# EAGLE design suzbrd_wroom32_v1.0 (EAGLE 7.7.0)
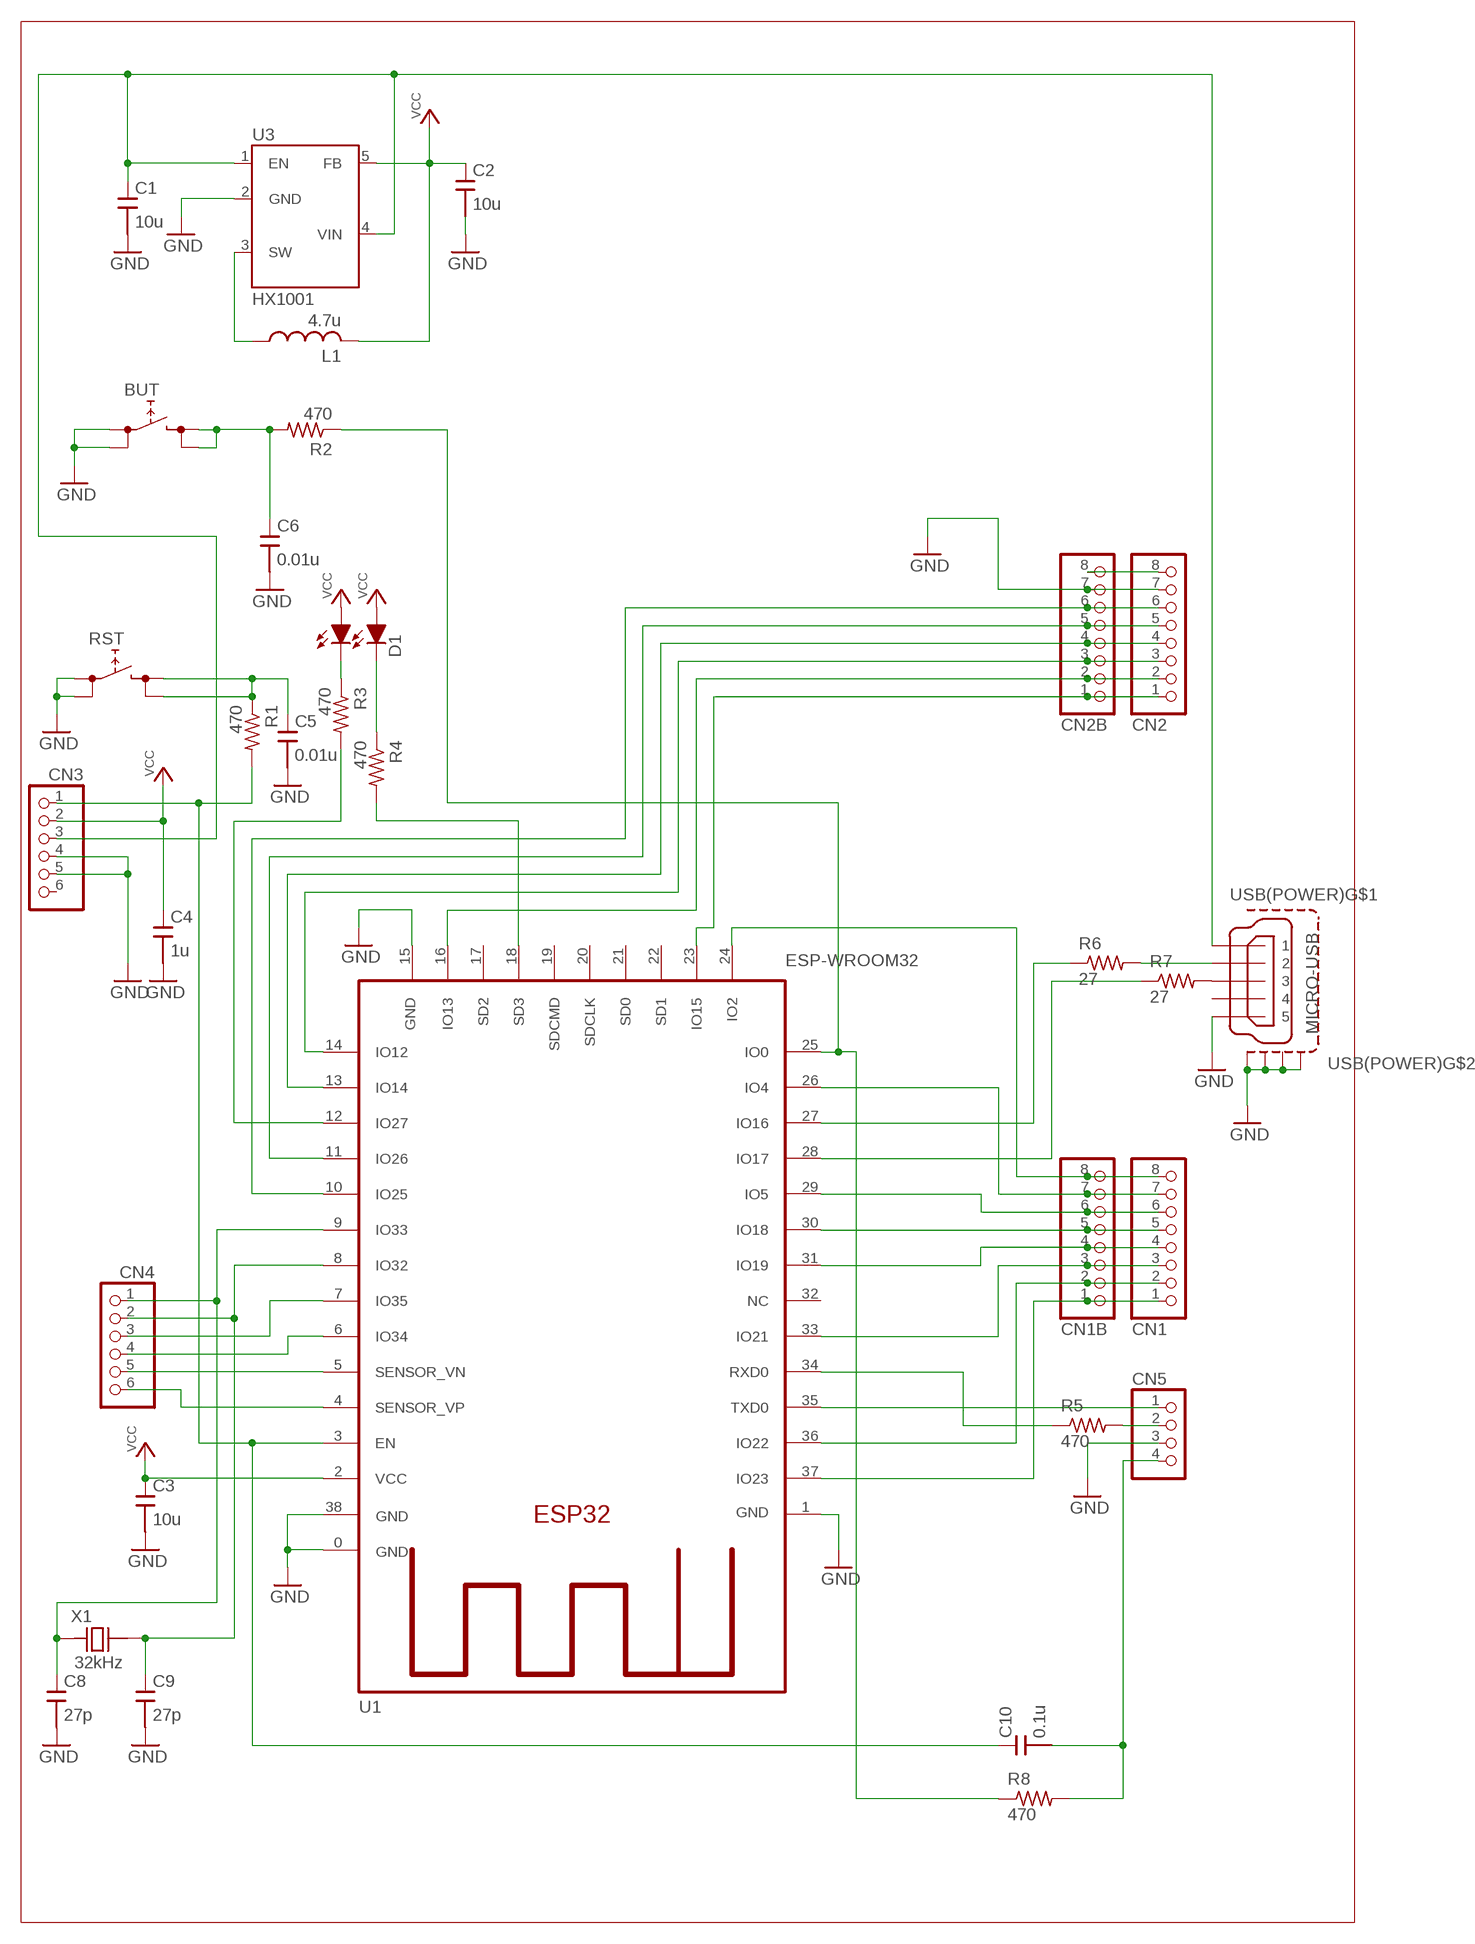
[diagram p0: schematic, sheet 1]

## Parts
BUT  TACTSWSMD+  [TACTSW/SMD+]
C1  10u  C/SMDC2012  [C2012]
C2  10u  C/SMDC2012  [C2012]
C3  10u  C/SMDC2012  [C2012]
C4  1u  C/SMDC2012  [C2012]
C5  0.01u  C/SMDC2012  [C2012]
C6  0.01u  C/SMDC2012  [C2012]
C8  27p  C/SMDC2012  [C2012]
C9  27p  C/SMDC2012  [C2012]
C10  0.1u  C/SMDC2012  [C2012]
CN1  PINHDR8  [PINHDR1X8]
CN1B  PINHDR81.0  [PINHDR1X8_1.0]
CN2  PINHDR8  [PINHDR1X8]
CN2B  PINHDR81.0  [PINHDR1X8_1.0]
CN3  PINHDR61.0  [PINHDR1X6_1.0]
CN4  PINHDR61.0  [PINHDR1X6_1.0]
CN5  CONN4N  [PINHDR1X4]
D1  SEC2XX4  [LED3025]
L1  4.7u  L/SMDNRG4026  [NRG4026]
R1  470  R/SMDR2012  [R2012]
R2  470  R/SMDR2012  [R2012]
R3  470  R/SMDR2012  [R2012]
R4  470  R/SMDR2012  [R2012]
R5  470  R/SMDR2012  [R2012]
R6  27  R/SMDR2012  [R2012]
R7  27  R/SMDR2012  [R2012]
R8  470  R/SMDR2012  [R2012]
RST  TACTSWSMD+  [TACTSW/SMD+]
U1  ESP-WROOM32  [ESP-WROOM32]
U3  HX1001  [SOT235]
USB(POWER)  MICRO-USB  [ZX62R]
X1  32kHz  CRYSTALFC255  [FC255]

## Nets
5V: C1.1 CN3.3 U3.1(EN) U3.4(VIN) USB(POWER).1
EN: C10.1 CN3.1 R1.2 U1.3(EN)
GND: BUT.1 BUT.2 C1.2 C2.2 C3.2 C4.2 C5.2 C6.2 C8.2 C9.2 CN2.7 CN2B.7 CN3.4 CN3.5 CN5.3 RST.1 RST.2 U1.0(GND) U1.1(GND) U1.15(GND) U1.38(GND) U3.2(GND) USB(POWER).5 USB(POWER).M1(S1) USB(POWER).M2(S2) USB(POWER).M3(S3) USB(POWER).M4(S4)
IO0: R2.1 R8.1 U1.25(IO0)
IO2: CN1.8 CN1B.8 U1.24(IO2)
IO4: CN1.7 CN1B.7 U1.26(IO4)
IO5: CN1.6 CN1B.6 U1.29(IO5)
IO12: CN2.3 CN2B.3 U1.14(IO12)
IO13: CN2.2 CN2B.2 U1.16(IO13)
IO14: CN2.4 CN2B.4 U1.13(IO14)
IO15: CN2.1 CN2B.1 U1.23(IO15)
IO16: R6.1 U1.27(IO16)
IO17: R7.1 U1.28(IO17)
IO18: CN1.5 CN1B.5 U1.30(IO18)
IO19: CN1.4 CN1B.4 U1.31(IO19)
IO21: CN1.3 CN1B.3 U1.33(IO21)
IO22: CN1.2 CN1B.2 U1.36(IO22)
IO23: CN1.1 CN1B.1 U1.37(IO23)
IO25: CN2.6 CN2B.6 U1.10(IO25)
IO26: CN2.5 CN2B.5 U1.11(IO26)
IO27: R3.2 U1.12(IO27)
IO32: C9.1 CN4.2 U1.8(IO32) X1.2
IO33: C8.1 CN4.1 U1.9(IO33) X1.1
IO34: CN4.4 U1.6(IO34)
IO35: CN4.3 U1.7(IO35)
N$1: R7.2 USB(POWER).3
N$3: CN5.2 R5.2
N$4: C10.2 CN5.4 R8.2
N$21: C5.1 R1.1 RST.3 RST.4
N$25: D1.2(C1) R3.1
N$26: D1.1(C0) R4.1
N$28: R4.2 U1.18(SD3)
N$32: R6.2 USB(POWER).2
N$36: CN2.8 CN2B.8
N$37: BUT.3 BUT.4 C6.1 R2.2
RXD0: R5.1 U1.34(RXD0)
SW: L1.1 U3.3(SW)
TXD0: CN5.1 U1.35(TXD0)
VCC: C2.1 C3.1 C4.1 CN3.2 D1.3(A1) D1.4(A0) L1.2 U1.2(VCC) U3.5(FB)
VN: CN4.5 U1.5(SENSOR_VN)
VP: CN4.6 U1.4(SENSOR_VP)
Unconnected: CN3.6 U1.17(SD2) U1.19(SDCMD) U1.20(SDCLK) U1.21(SD0) U1.22(SD1) U1.32(NC) USB(POWER).4

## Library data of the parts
BUT RST = SRT162-010:TACTSW: 4pin tactsw (1,2 - 3,4)
C1-C6 C8-C10 = SRT162-010:C/SMD
CN1 CN1B CN2 CN2B = SRT162-010:PINHDR8
CN3 CN4 = SRT162-010:PINHDR6
CN5 = SRT162-010:CONN4: connector 4
D1 = SRT162-010:SEC2XX4
L1 = SRT162-010:L/SMD: VLF4012AT
R1-R8 = SRT162-010:R/SMD
U1 = SRT162-020:ESP-WROOM32
U3 = SRT162-010:HX1001
USB(POWER) = SRT162-020:MICRO-USB
X1 = SRT162-020:CRYSTAL

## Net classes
1 Power: width 0.381 mm, clearance 0.203 mm to class 0

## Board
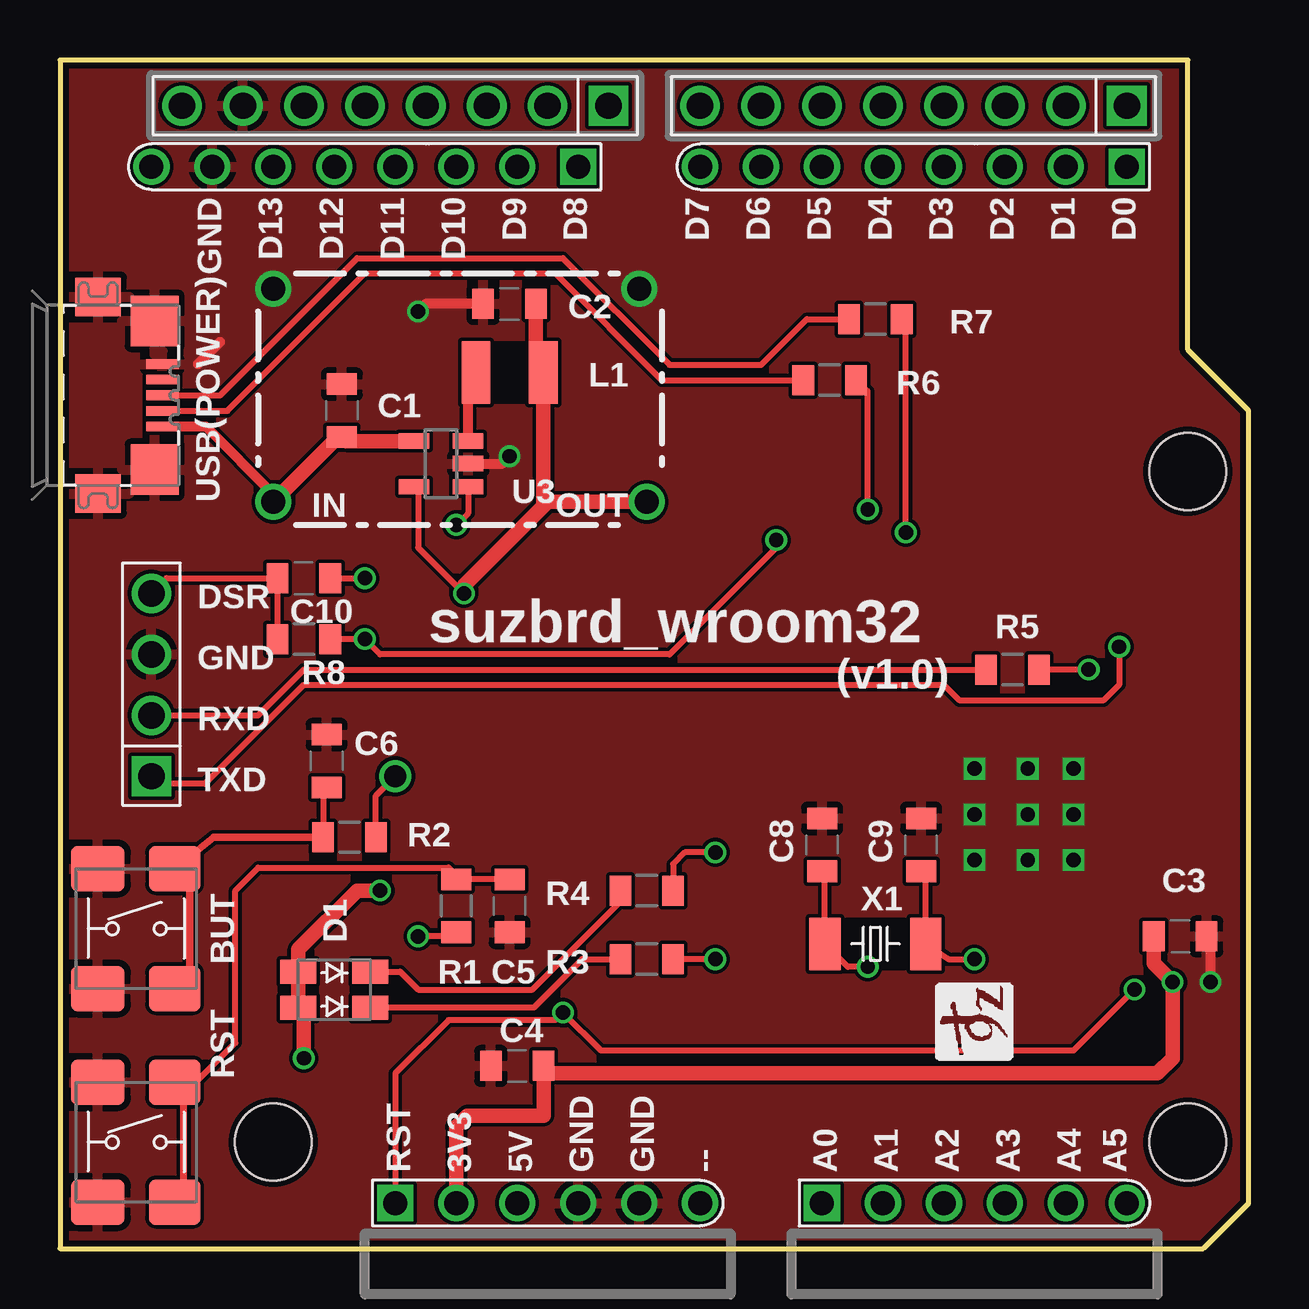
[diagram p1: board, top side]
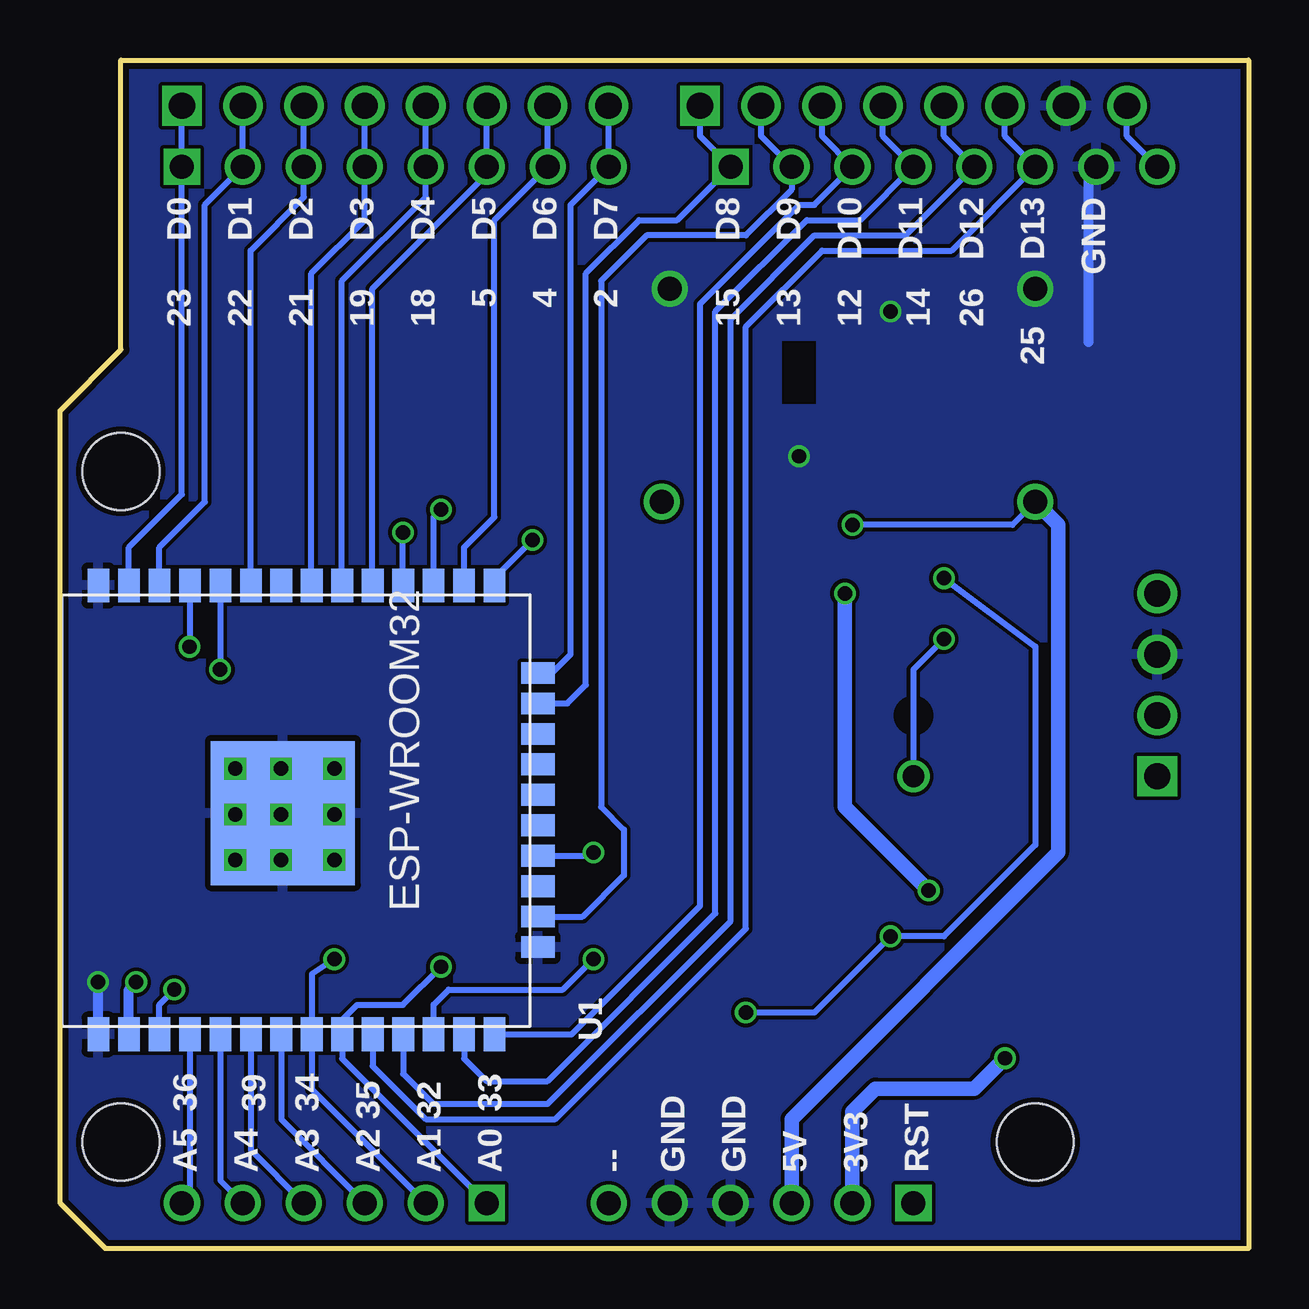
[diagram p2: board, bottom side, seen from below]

Size 49.53 x 49.53 mm. Coordinates in mm from the lower left corner, seen from the top.
Outline: 0,0 47.62,0 49.53,1.91 49.53,34.93 46.99,37.47 46.99,49.53 0,49.53 0,0
Copper layers (1*16): Top 0.035mm / dielectric 1.5mm / Bottom 0.035mm
Design rules "SeeedStudio": minimum track width 6mil, minimum drill 12mil, track to track 6mil, track to pad 6mil, pad to pad 6mil, via to via 6mil, smd to smd 0mil, copper to edge 10mil, drill to drill 10mil, minimum pad ring 10mil, minimum via ring 6mil, stop-mask expansion 2mil, vias tented up to drill 25mil, thermal gap 10mil
Holes 3.2 mm at 46.99,4.45 46.99,32.39 8.89,4.45
bRestrict: area 13.7,21.9 to 14.3,22.5
vRestrict: area 1.9,41.9 to 45.7,44.5; area 12.7,3.2 to 44.4,5.1

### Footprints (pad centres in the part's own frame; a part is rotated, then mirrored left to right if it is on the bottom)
TACTSW/SMD+ = smd 2.25 x 1.9: 1 -1.6,2.5; 2 -1.6,-2.5 | smd 2.15 x 1.9: 3 1.6,2.5; 4 1.6,-2.5
C2012 = smd 0.9 x 1.25: 1 -1.1,0; 2 1.1,0
PINHDR1X8 = drill 1.1 square: 1 -8.89,0 | drill 1.1: 2 -6.35,0; 3 -3.81,0; 4 -1.27,0; 5 1.27,0; 6 3.81,0; 7 6.35,0; 8 8.89,0
PINHDR1X8_1.0 = drill 1 square: 1 -8.89,0 | drill 1: 2 -6.35,0; 3 -3.81,0; 4 -1.27,0; 5 1.27,0; 6 3.81,0; 7 6.35,0; 8 8.89,0
PINHDR1X6_1.0 = drill 1 square: 1 -6.35,0 | drill 1: 2 -3.81,0; 3 -1.27,0; 4 1.27,0; 5 3.81,0; 6 6.35,0
PINHDR1X4 = drill 1.1 square: 1 -3.81,0 | drill 1.1: 2 -1.27,0; 3 1.27,0; 4 3.81,0
LED3025 = smd 1.5 x 1: 1 1.5,0.75; 2 1.5,-0.75; 3 -1.5,-0.75; 4 -1.5,0.75
NRG4026 = smd 1.2 x 2.6: 1 -1.4,0; 2 1.4,0
R2012 = smd 0.9 x 1.25: 1 -1.1,0; 2 1.1,0
ESP-WROOM32 = smd 6 x 6: 0 9.9,12.3 | smd 1.4 x 0.9: 1 0.68,19.99; 2 0.68,18.72; 3 0.68,17.45; 4 0.68,16.18; 5 0.68,14.91; 6 0.68,13.64; 7 0.68,12.37; 8 0.68,11.1; 9 0.68,9.83; 10 0.68,8.56; 11 0.68,7.29; 12 0.68,6.02; 13 0.68,4.75; 14 0.68,3.48; 25 19.38,3.48; 26 19.38,4.75; 27 19.38,6.02; 28 19.38,7.29; 29 19.38,8.56; 30 19.38,9.83; 31 19.38,11.1; 32 19.38,12.37; 33 19.38,13.64; 34 19.38,14.91; 35 19.38,16.18; 36 19.38,17.45; 37 19.38,18.72; 38 19.38,19.99 | smd 0.9 x 1.4: 15 4.31,1.68; 16 5.58,1.68; 17 6.85,1.68; 18 8.12,1.68; 19 9.39,1.68; 20 10.66,1.68; 21 11.93,1.68; 22 13.2,1.68; 23 14.47,1.68; 24 15.74,1.68
SOT235 = smd 0.635 x 1.27: 1 -0.95,-1.125; 2 0.013,-1.135; 3 0.95,-1.125; 4 0.95,1.125; 5 -0.95,1.125
ZX62R = smd 1.35 x 0.4: 1 2.675,-1.3; 2 2.675,-0.65; 3 2.675,0; 4 2.675,0.65; 5 2.675,1.3 | smd 1.9 x 1.6: M1 0,-4.1; M2 0,4.1 | smd 2 x 2.1: M3 2.35,3.1; M4 2.35,-3.1
FC255 = smd 1.3 x 2.2: 1 2.1,0; 2 -2.1,0

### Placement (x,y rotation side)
BUT  3.18,13.34 0 top
C1  11.75,34.93 90 top
C2  18.73,39.37 180 top
C3  46.67,13.02 0 top
C4  19.05,7.62 180 top
C5  18.73,14.29 270 top
C6  11.11,20.32 90 top
C8  31.75,16.83 90 top
C9  35.88,16.83 90 top
C10  10.16,27.94 180 top
CN1  35.56,47.62 180 top
CN1B  35.56,45.09 180 top
CN2  13.97,47.62 180 top
CN2B  12.7,45.09 180 top
CN3  20.32,1.91 0 top
CN4  38.1,1.91 0 top
CN5  3.81,23.5 90 top
D1  11.43,10.8 0 top
L1  18.73,36.51 0 top
R1  16.51,14.29 270 top
R2  12.07,17.14 180 top
R3  24.45,12.07 0 top
R4  24.45,14.92 0 top
R5  39.69,24.13 180 top
R6  32.07,36.2 180 top
R7  33.97,38.73 180 top
R8  10.16,25.4 180 top
RST  3.18,4.45 0 top
U1  27.94,8.25 90 bottom
U3  15.88,32.7 90 top
USB(POWER)  1.59,35.56 0 top
X1  33.97,12.7 180 top

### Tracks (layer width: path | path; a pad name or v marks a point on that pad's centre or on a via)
5V  (via drill 0.6, 1)
  Top 0.254: U3.1 17,30.65 v16.51,30.16
  Top 0.406: v8.89,31.11 8.89,31.43 6.06,34.26 USB(POWER).1
  Top 0.61: v8.89,31.11 11.6,33.83 C1.1 11.92,33.65 U3.4
  Bottom 0.254: v8.89,31.11 9.84,30.16 v16.51,30.16
  Bottom 0.61: CN3.3 19.05,5.4 7.94,16.51 7.94,30.16 v8.89,31.11
EN  (via drill 0.6)
  Top 0.254: 13.93,1.95 CN3.1 13.97,7.3 16.19,9.52 20.64,9.52 v20.96,9.84 22.54,8.25 42.23,8.25 v44.77,10.8 | R1.2 16.34,13.02 v14.92,13.02 | C10.1 v12.7,27.94
  Bottom 0.254: U1.3 45.39,10.17 v44.77,10.8 | v20.96,9.84 18.1,9.84 v14.92,13.02 12.7,13.02 8.89,16.83 8.89,25.08 v12.7,27.94
  Bottom 0.3: CN3.1
GND  (via drill 0.6, 1)
  Top 0.406: v47.94,11.11 47.94,12.85 C3.2 | 5.74,36.86 6.67,37.78 | U3.2 18.43,32.72 v18.73,33.02 | C2.2 15.24,39.37 v14.92,39.05
  Bottom 0.406: U1.1 47.93,11.1 v47.94,11.11 | 6.67,37.78 6.67,44.77 CN2B.7
  other vias: 42.23,16.19 42.23,20 38.1,20 38.1,16.19 40.32,18.1 40.32,16.19 38.1,18.1 42.23,18.1 40.32,20 8.89,40.01 24.13,40.01
  pour Bottom: -0.64,50.17 52.07,50.17 52.07,-3.17 -0.64,-3.17
  pour Top: -1.27,50.8 53.34,50.8 53.34,-3.81 -1.27,-3.81
IO0  (via drill 0.6, 0.9)
  Top 0.254: R8.1 v12.7,25.4 13.34,24.77 25.4,24.77 29.84,29.21 v29.84,29.53 | R2.1 13.17,18.88 v13.97,19.68
  Bottom 0.254: U1.25 31.42,27.95 v29.84,29.53 | v12.7,25.4 13.97,24.13 v13.97,19.68
IO2
  Bottom 0.254: U1.24 29.03,24 28.26,24.77 28.26,43.5 CN1B.8 CN1.8
IO4
  Bottom 0.254: U1.26 32.69,29.22 31.43,30.48 31.43,42.86 CN1B.7 CN1.7
IO5
  Bottom 0.254: U1.29 36.51,27.65 36.51,40.01 31.75,44.77 CN1B.6 CN1.6
IO12
  Bottom 0.254: U1.14 28.21,8.93 22.86,14.29 22.86,39.37 18.73,43.5 18.1,43.5 CN2B.3 17.78,46.36 CN2.3
IO13
  Bottom 0.254: U1.16 27.76,13.84 26.04,15.56 26.04,17.46 26.99,18.41 26.99,40.32 25.08,42.23 20.96,42.23 19.05,44.13 CN2B.2 20.32,46.36 CN2.2
IO14
  Bottom 0.254: U1.13 32.69,7.92 31.75,6.99 29.21,6.99 22.23,13.97 22.23,39.05 18.41,42.86 16.19,42.86 CN2B.4 15.24,46.36 CN2.4
IO15
  Bottom 0.254: U1.23 28.39,22.72 27.62,23.5 27.62,40.64 25.4,42.86 23.81,42.86 CN2B.1 22.86,46.36 CN2.1
IO16  (via drill 0.6)
  Top 0.254: v33.65,30.8 33.65,35.73 R6.1
  Bottom 0.254: U1.27 33.96,30.49 v33.65,30.8
IO17  (via drill 0.6)
  Top 0.254: v35.24,29.85 35.24,38.57 R7.1
  Bottom 0.254: U1.28 35.24,27.65 v35.24,29.85
IO18
  Bottom 0.254: U1.30 37.78,27.65 37.78,40.32 34.29,43.82 CN1B.5 CN1.5
IO19
  Bottom 0.254: U1.31 39.05,27.65 39.05,40.64 36.83,42.86 CN1B.4 CN1.4
IO21
  Bottom 0.254: U1.33 41.59,27.65 41.59,41.59 39.37,43.82 CN1B.3 CN1.3
IO22
  Bottom 0.254: CN1.2 CN1B.2 43.5,43.5 43.5,31.11 45.39,29.22 U1.36
IO23
  Bottom 0.254: U1.37 46.66,29.22 44.45,31.43 CN1B.1 CN1.1
IO25
  Bottom 0.254: U1.10 36.5,7.61 34.29,5.4 28.89,5.4 20.96,13.34 20.96,38.42 17.78,41.59 12.38,41.59 CN2B.6 10.16,46.36 CN2.6
IO26
  Bottom 0.254: U1.11 35.23,7.29 33.97,6.03 29.21,6.03 21.59,13.65 21.59,38.73 18.1,42.23 14.29,42.23 CN2B.5 12.7,46.36 CN2.5
IO27  (via drill 0.6)
  Top 0.254: v27.3,12.07 R3.2
  Bottom 0.254: U1.12 33.96,10.17 33.34,10.8 28.57,10.8 v27.3,12.07
IO32  (via drill 0.6)
  Top 0.254: v38.1,12.07 37.02,12.07 X1.2 36.07,15.53 C9.1
  Bottom 0.254: CN4.2 39.04,6.66 U1.8 39.04,11.44 v38.1,12.07
IO33  (via drill 0.6)
  Top 0.254: v33.65,11.75 32.82,11.75 X1.1 31.87,15.61 C8.1
  Bottom 0.254: CN4.1 37.77,7.92 U1.9 37.77,9.54 37.15,10.16 35.24,10.16 v33.65,11.75
IO34
  Bottom 0.254: U1.6 41.58,4.12 CN4.4
IO35
  Bottom 0.254: U1.7 40.31,5.39 CN4.3
N$1
  Top 0.254: USB(POWER).3 6.67,35.56 12.38,41.28 20.96,41.28 25.4,36.83 29.21,36.83 31.11,38.73 R7.2
N$3
  Top 0.254: CN5.2 8.26,22.22 10.16,24.13 R5.2
N$4
  Top 0.254: CN5.4 4.45,27.94 C10.2 R8.2
N$21
  Top 0.254: 5.16,6.27 5.16,6.43 7.3,8.57 7.3,14.92 8.26,15.88 16.19,15.88 16.83,15.24 16.66,15.24 R1.1 C5.1
  Top 0.3: RST.4 5.16,2.14 5.16,6.27 RST.3
N$25
  Top 0.254: D1.2 19.74,10.05 21.76,12.07 R3.1
N$26
  Top 0.254: D1.1 14.17,11.55 14.92,10.8 19.68,10.8 23.35,14.46 R4.1
N$28  (via drill 0.6)
  Top 0.254: v27.3,16.51 26.04,16.51 25.55,16.02 R4.2
  Bottom 0.254: U1.18 27.44,16.38 v27.3,16.51
N$32
  Top 0.254: R6.2 25.08,36.2 20.64,40.64 12.7,40.64 6.97,34.91 USB(POWER).2
N$36
  Bottom 0.254: CN2B.8 5.08,46.36 CN2.8
N$37
  Top 0.152: BUT.4 4.84,10.88 5.32,10.88 5.32,11.03 5.4,11.11
  Top 0.254: C6.1 10.96,19.07 R2.2
  Top 0.305: R2.2 6.4,17.14 BUT.3 5.4,15.84 5.4,11.11
RXD0  (via drill 0.6)
  Top 0.254: v42.86,24.13 R5.1
  Bottom 0.254: U1.34 42.85,24.14 v42.86,24.13
SW
  Top 0.406: U3.3 17,36.18 L1.1
TXD0  (via drill 0.6)
  Top 0.254: v44.13,25.08 44.13,23.5 43.5,22.86 37.46,22.86 36.83,23.5 10.16,23.5 6.03,19.37 4.13,19.37 CN5.1
  Bottom 0.254: U1.35 v44.12,25.09 v44.13,25.08
VCC  (via drill 0.6, 1)
  Top 0.254: U3.5 14.92,31.58 14.92,29.21 v16.83,27.3
  Top 0.406: C4.1 20.47,7.3 | 10.16,9.82 D1.3 | 19.83,36.81 L1.2
  Top 0.61: C3.1 45.57,11.89 v46.35,11.11 46.35,7.94 45.72,7.3 20.47,7.3 | C4.1 20.15,5.55 16.98,5.55 16.51,5.08 CN3.2 | v10.16,7.94 10.16,9.82 | D1.3 D1.4 9.93,12.47 12.38,14.92 v13.34,14.92 | C2.1 19.83,36.81 | L1.2 20.13,30.93 | v24.45,31.11 20.32,31.11 20.13,30.93 | 20.13,30.93 16.83,27.62 v16.83,27.3
  Bottom 0.406: U1.2 46.66,10.81 v46.35,11.11
  Bottom 0.61: CN3.2 16.51,5.72 15.56,6.67 11.43,6.67 v10.16,7.94 | v13.34,14.92 16.83,18.41 v16.83,27.3
VN
  Bottom 0.254: U1.5 42.85,2.84 CN4.5
VP
  Bottom 0.254: U1.4 44.12,2.24 CN4.6

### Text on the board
tPlace: GND | D13 | D12 | D11 | D10 | D9 | D8 | D7 | D6 | D5 | D4 | D3 | D2 | D1 | D0 | IN | OUT | DSR | suzbrd_wroom32 | (v1.0) | GND | RXD | TXD | RST | 3V3 | 5V | GND | GND | -- | A0 | A1 | A2 | A3 | A4 | A5
bPlace: GND | D13 | D12 | D11 | D10 | D9 | D8 | D7 | D6 | D5 | D4 | D3 | D2 | D1 | D0 | 26 | 14 | 12 | 13 | 15 | 2 | 4 | 5 | 18 | 19 | 21 | 22 | 23 | 25 | 33 | 32 | 35 | 34 | 39 | 36 | RST | 3V3 | 5V | GND | GND | -- | A0 | A1 | A2 | A3 | A4 | A5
